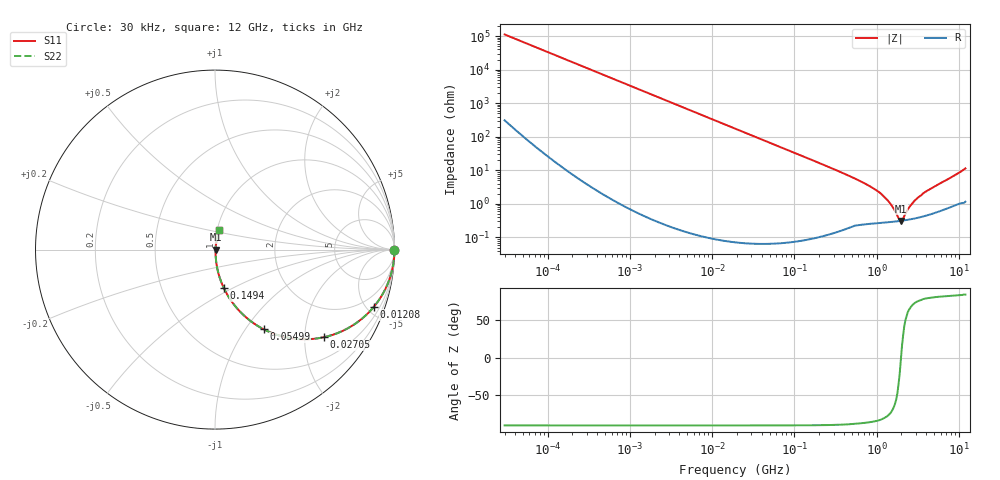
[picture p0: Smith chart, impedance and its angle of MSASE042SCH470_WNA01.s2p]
! MSASE042SCH470_WNA01  S-PARAMETER MODEL  ( General Type )
! Model Generated by TAIYO YUDEN Corporation (http://www.ty-top.com)
! Version 3.0
! TAIYO YUDEN Control No. 120810
! Copyright(c) 2007 TAIYO YUDEN CO.,LTD. All Rights Reserved.
! Product Description (link to TY-COMPAS)
! https://ds.yuden.co.jp/TYCOMPAS/or/detail?pn=MSASE042SCH470JWNA01&u=M
! Products Name : Multilayer Ceramic Capacitors
! Characteristics :
!  Capacitance : 47 pF , Rated Voltage : 16V , TCC : CH / C0H
!  Case Size : 0.4 x 0.2 / 0.016 x 0.008 [mm/inch] , Thickness : 0.2 / 0.008 [mm/inch]
!  (Conditions: Temperature = 25 degC , DC Bias Current/Voltage = 0A / 0V)
! External Node Assignments :
!  1  o---| |---o  2
! GND o---------o GND
! Frequency Range : 0.03MHz  -  12000MHz  [ 401 STEP ]
# MHz S RI R 50
! Freq[MHz].  S11 Real  S11 Imag  S21 Real  S21 Imag  S12 Real  S12 Imag  S22 Real  S22 Imag
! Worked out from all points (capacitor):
!   401 points, 30 kHz to 12 GHz, reference 50 ohm
!   read as one part in series: C = 47.4 pF near 32 kHz
!   lowest |Z| = 314 mohm at 1.972 GHz (marker M1)
!   series resonance near 1.978 GHz, so ESL is about 140 pH
!   S11 on the Smith chart (normalised r, x): 30 kHz: open; 12.08 MHz: 1.00, -5.56; 27.05 MHz: 1.00, -2.48; 54.99 MHz: 1.00, -1.22; 149.4 MHz: 1.00, -0.45; 12 GHz: 1.02, +0.23
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0.03  1 -0.000894  3.27e-06 0.000894  3.27e-06 0.000894  1 -0.000894
0.260295  0.9999 -0.00776  6.31e-05 0.00776  6.31e-05 0.00776  0.9999 -0.00776
2.258455  0.9955 -0.067  0.00452 0.067  0.00452 0.067  0.9955 -0.067
5.39449  0.9748 -0.1567  0.0252 0.1567  0.0252 0.1567  0.9748 -0.1567
12.08034  0.8852 -0.3186  0.1148 0.3186  0.1148 0.3186  0.8852 -0.3186
18.97367  0.7576 -0.4283  0.2424 0.4283  0.2424 0.4283  0.7576 -0.4283
27.05253  0.606 -0.4884  0.394 0.4884  0.394 0.4884  0.606 -0.4884
38.57132  0.4307 -0.4948  0.5693 0.4948  0.5693 0.4948  0.4307 -0.4948
54.99475  0.2712 -0.4441  0.7288 0.4441  0.7288 0.4441  0.2712 -0.4441
86.37604  0.1312 -0.3367  0.8688 0.3367  0.8688 0.3367  0.1312 -0.3367
149.4448  0.0482 -0.2123  0.9518 0.2123  0.9518 0.2123  0.0482 -0.2123
164.6252  0.0402 -0.1941  0.9598 0.1941  0.9598 0.1941  0.0402 -0.1941
749.4426  0.00395 -0.0382  0.9961 0.0382  0.9961 0.0382  0.00395 -0.0382
1068.55  0.00318 -0.0222  0.9968 0.0222  0.9968 0.0222  0.00318 -0.0222
1428.372  0.00297 -0.0107  0.997 0.0107  0.997 0.0107  0.00297 -0.0107
1848.769  0.00307 -0.00211  0.9969 0.00211  0.9969 0.00211  0.00307 -0.00211
1971.936  0.00312 -9.07e-05  0.9969 9.07e-05  0.9969 9.07e-05  0.00312 -9.07e-05
2103.309  0.0032 0.00188  0.9968 -0.00188  0.9968 -0.00188  0.0032 0.00188
2392.896  0.00339 0.00601  0.9966 -0.00601  0.9966 -0.00601  0.00339 0.00601
2722.352  0.00365 0.00983  0.9963 -0.00983  0.9963 -0.00983  0.00365 0.00983
3639.072  0.00457 0.0197  0.9954 -0.0197  0.9954 -0.0197  0.00457 0.0197
12000  0.0238 0.1096  0.9762 -0.1096  0.9762 -0.1096  0.0238 0.1096
